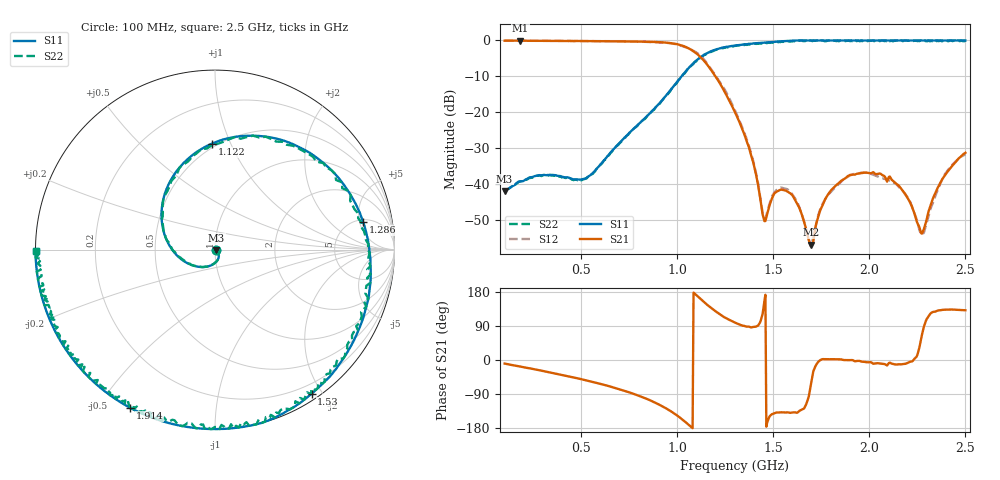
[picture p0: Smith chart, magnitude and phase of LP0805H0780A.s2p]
!	AVX	THIN	FILM	OPERATION
!	LP0805	High	Performance	Low	Pass	Filter	P/N	LP0805H0780ASTR
!	25	June	2017
#	MHz	S	dB	R	50
!	Frq	S11(dB)	S11(deg)	S21(dB)	S21(deg)	S12(dB)	S12(deg)	S22(dB)	S22(deg)
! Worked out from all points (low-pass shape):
!   501 points, 100 MHz to 2.5 GHz, reference 50 ohm
!   highest |S21| = -0.02 dB at 181.6 MHz (marker M1); lowest = -56.8 dB at 1.698 GHz (marker M2)
!   |S21| within 3 dB of the highest: start of sweep to 1.084 GHz
!   lowest |S11| = -41.9 dB at 100 MHz (marker M3), VSWR 1.02, Z = 50.7 - j0.452 ohm
!   |S11| at or under -10 dB: start of sweep to 1.021 GHz
!   |S22| runs from -42.1 to 0.0 dB; largest |S21 - S12| = 0.043
!   S11 on the Smith chart (normalised r, x): 100 MHz: 1.01, -0.01; 1.122 GHz: 0.47, +0.85; 1.286 GHz: 5.43, +5.67; 1.53 GHz: 0.08, -1.87; 1.914 GHz: 0.00, -0.60; 2.5 GHz: -0.00, -0.00
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100  -41.88 -33.6  -0.07 -9.4  -0.06 -9.5  -42.08 -33.8
181.6  -39.19 -56.2  -0.02 -17.3  -0.05 -17.7  -39.19 -56.3
503.2  -38.62 -71.0  -0.16 -51.1  -0.15 -51.3  -38.82 -71.0
901.6  -17.76 -131.9  -0.46 -116.9  -0.53 -116.5  -17.76 -132.1
1026.4  -9.67 153.8  -1.45 -157.3  -1.58 -156.0  -9.77 153.8
1122.4  -4.58 91.8  -4.73 160.3  -4.37 162.4  -4.68 91.5
1189.6  -2.71 53.1  -9.30 131.9  -9.05 133.2  -2.81 53.1
1285.6  -1.52 10.6  -18.35 102.1  -17.78 100.9  -1.62 10.4
1300  -1.41 5.4  -19.93 98.7  -19.46 97.3  -1.51 5.4
1386.4  -0.89 -21.7  -32.41 86.2  -31.79 84.5  -0.99 -21.9
1453.6  -0.58 -39.1  -50.27 157.3  -49.58 156.0  -0.58 -39.3
1530.4  -0.29 -56.2  -41.68 -138.5  -41.11 -141.6  -0.29 -56.4
1607.2  -0.05 -71.2  -43.80 -138.2  -43.47 -143.7  -0.25 -71.3
1698.4  0.00 -87.0  -56.82 -55.7  -57.07 -57.0  -0.10 -87.0
1703.2  0.00 -87.8  -56.38 -42.7  -55.73 -46.0  -0.20 -87.9
1780  0.00 -99.6  -43.22 2.0  -43.21 -5.9  -0.10 -99.6
1914.4  0.00 -118.2  -37.32 -0.7  -37.21 -4.7  0.00 -118.2
2101.6  0.00 -140.7  -37.96 -8.0  -38.88 -10.8  0.00 -140.9
2202.4  0.00 -151.3  -44.13 -7.0  -43.93 -9.7  -0.10 -151.4
2274.4  0.00 -158.6  -53.72 67.9  -54.04 58.7  -0.10 -158.7
2389.6  0.00 -169.5  -37.78 132.7  -37.53 135.8  0.00 -169.7
2500  0.00 -179.4  -31.24 131.2  -31.70 125.4  0.00 -179.5
